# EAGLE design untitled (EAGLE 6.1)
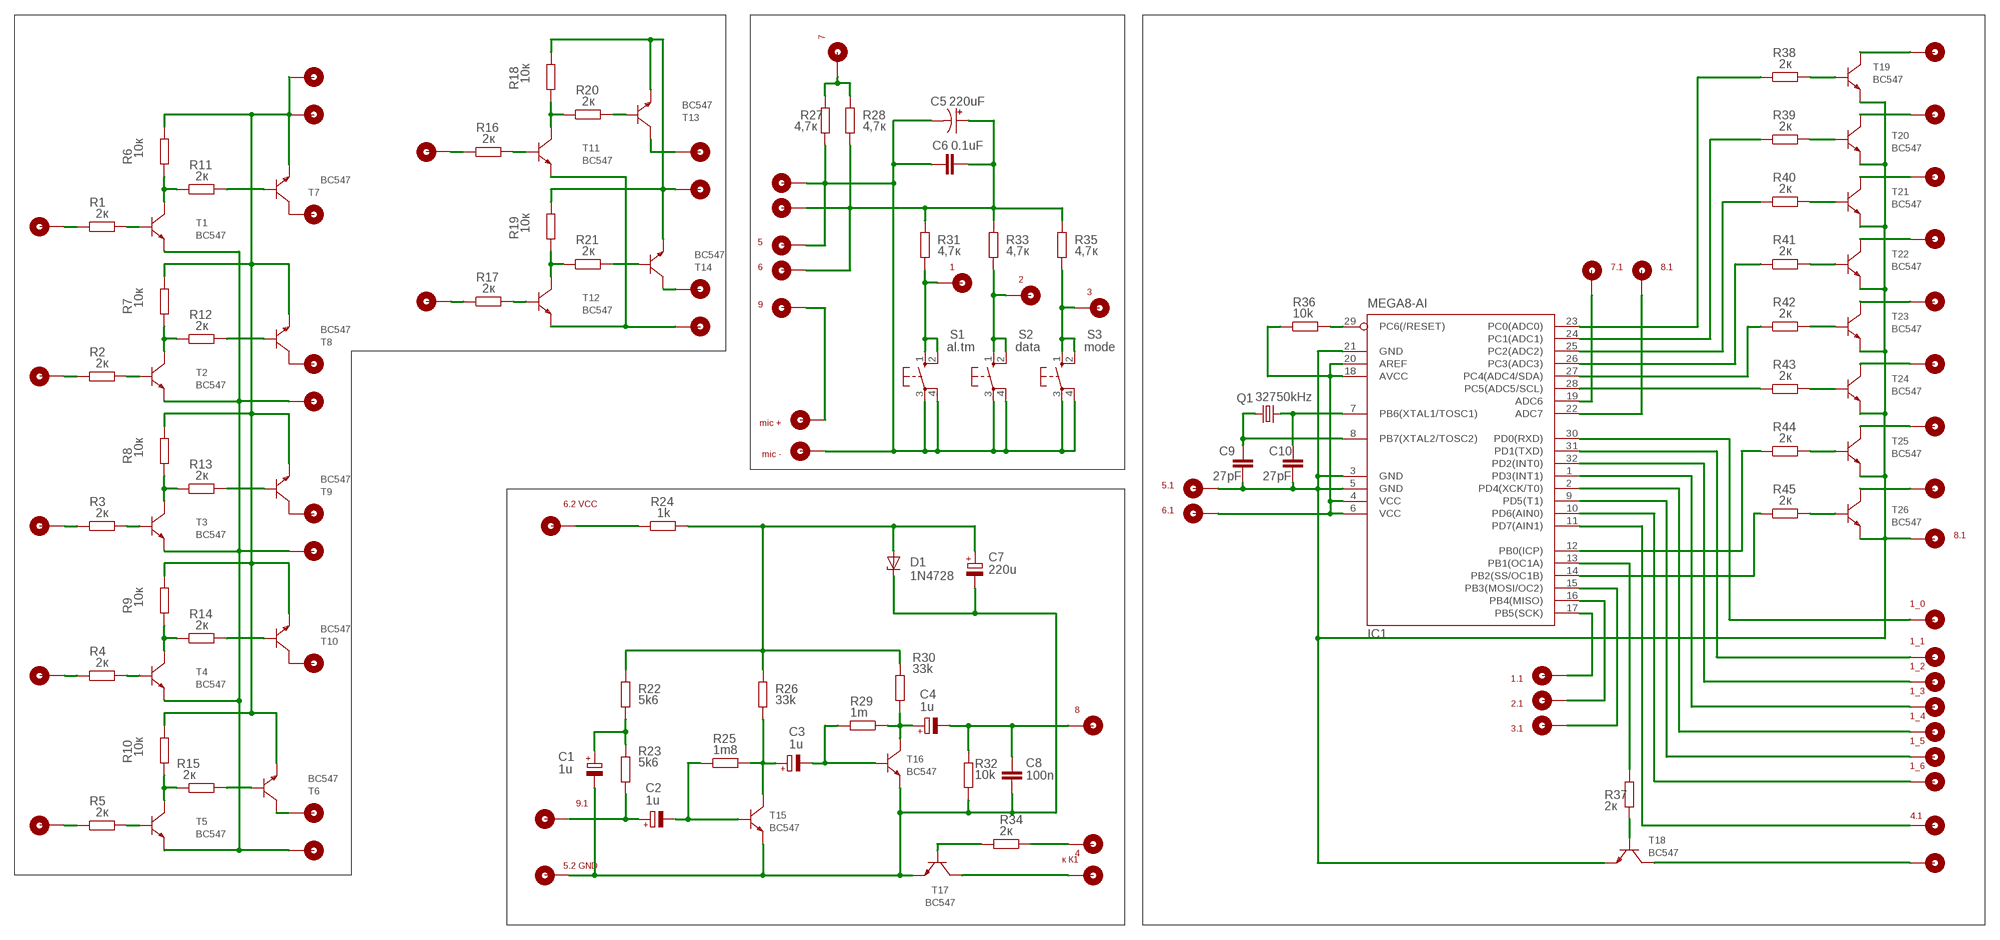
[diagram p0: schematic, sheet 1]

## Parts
1  1_0  PIN_1  [PIN_1]
2  1_1  PIN_1  [PIN_1]
3  1_2  PIN_1  [PIN_1]
C1  1u  CPOL-EUE2.5-6  [E2,5-6]
C2  1u  CPOL-EUE2.5-6  [E2,5-6]
C3  1u  CPOL-EUE2.5-6  [E2,5-6]
C4  1u  CPOL-EUE2.5-6  [E2,5-6]
C5  220uF  CPOL-US153CLV-0810  [153CLV-0810]
C6  0.1uF  C-EU050-024X044  [C050-024X044]
C7  220u  CPOL-EUE3.5-8  [E3,5-8]
C8  100n  C-EU050-024X044  [C050-024X044]
C9  27pF  C-EU050-024X044  [C050-024X044]
C10  27pF  C-EU050-024X044  [C050-024X044]
D1  1N4728  [DO41Z10]
IC1  MEGA8-AI  [TQFP32-08]
Q1  32750kHz  CRYSTALTC38H  [TC38H]
R1  2к  R-EU_0207/10  [0207/10]
R2  2к  R-EU_0207/10  [0207/10]
R3  2к  R-EU_0207/10  [0207/10]
R4  2к  R-EU_0207/10  [0207/10]
R5  2к  R-EU_0207/10  [0207/10]
R6  10к  R-EU_0207/10  [0207/10]
R7  10к  R-EU_0207/10  [0207/10]
R8  10к  R-EU_0207/10  [0207/10]
R9  10к  R-EU_0207/10  [0207/10]
R10  10к  R-EU_0207/10  [0207/10]
R11  2к  R-EU_0207/10  [0207/10]
R12  2к  R-EU_0207/10  [0207/10]
R13  2к  R-EU_0207/10  [0207/10]
R14  2к  R-EU_0207/10  [0207/10]
R15  2к  R-EU_0207/10  [0207/10]
R16  2к  R-EU_0207/10  [0207/10]
R17  2к  R-EU_0207/10  [0207/10]
R18  10к  R-EU_0207/10  [0207/10]
R19  10к  R-EU_0207/10  [0207/10]
R20  2к  R-EU_0207/10  [0207/10]
R21  2к  R-EU_0207/10  [0207/10]
R22  5k6  R-EU_0207/10  [0207/10]
R23  5k6  R-EU_0207/10  [0207/10]
R24  1k  R-EU_0207/10  [0207/10]
R25  1m8  R-EU_0207/10  [0207/10]
R26  33k  R-EU_0207/10  [0207/10]
R27  4,7к  R-EU_0207/10  [0207/10]
R28  4,7к  R-EU_0207/10  [0207/10]
R29  1m  R-EU_0207/10  [0207/10]
R30  33k  R-EU_0207/10  [0207/10]
R31  4,7к  R-EU_0207/10  [0207/10]
R32  10k  R-EU_0207/10  [0207/10]
R33  4,7к  R-EU_0207/10  [0207/10]
R34  2к  R-EU_0207/10  [0207/10]
R35  4,7к  R-EU_0207/10  [0207/10]
R36  10k  R-EU_0207/12  [0207/12]
R37  2к  R-EU_0207/10  [0207/10]
R38  2к  R-EU_0207/10  [0207/10]
R39  2к  R-EU_0207/10  [0207/10]
R40  2к  R-EU_0207/10  [0207/10]
R41  2к  R-EU_0207/10  [0207/10]
R42  2к  R-EU_0207/10  [0207/10]
R43  2к  R-EU_0207/10  [0207/10]
R44  2к  R-EU_0207/10  [0207/10]
R45  2к  R-EU_0207/10  [0207/10]
S1  al.tm  10-XX  [B3F-10XX]
S2  data  10-XX  [B3F-10XX]
S3  mode  10-XX  [B3F-10XX]
T1  BC547  [BC547]
T2  BC547  [BC547]
T3  BC547  [BC547]
T4  BC547  [BC547]
T5  BC547  [BC547]
T6  BC547  [BC547]
T7  BC547  [BC547]
T8  BC547  [BC547]
T9  BC547  [BC547]
T10  BC547  [BC547]
T11  BC547  [BC547]
T12  BC547  [BC547]
T13  BC547  [BC547]
T14  BC547  [BC547]
T15  BC547  [BC547]
T16  BC547  [BC547]
T17  BC547  [BC547]
T18  BC547  [BC547]
T19  BC547  [BC547]
T20  BC547  [BC547]
T21  BC547  [BC547]
T22  BC547  [BC547]
T23  BC547  [BC547]
T24  BC547  [BC547]
T25  BC547  [BC547]
T26  BC547  [BC547]
U$1  PIN_1  [PIN_1]
U$2  PIN_1  [PIN_1]
U$3  PIN_1  [PIN_1]
U$4  PIN_1  [PIN_1]
U$5  PIN_1  [PIN_1]
U$6  PIN_1  [PIN_1]
U$7  PIN_1  [PIN_1]
U$8  PIN_1  [PIN_1]
U$9  PIN_1  [PIN_1]
U$10  PIN_1  [PIN_1]
U$11  PIN_1  [PIN_1]
U$12  PIN_1  [PIN_1]
U$13  PIN_1  [PIN_1]
U$14  PIN_1  [PIN_1]
U$15  PIN_1  [PIN_1]
U$16  PIN_1  [PIN_1]
U$17  PIN_1  [PIN_1]
U$18  9.1  PIN_1  [PIN_1]
U$19  5.2 GND  PIN_1  [PIN_1]
U$20  6.2 VCC  PIN_1  [PIN_1]
U$21  PIN_1  [PIN_1]
U$22  PIN_1  [PIN_1]
U$23  PIN_1  [PIN_1]
U$24  PIN_1  [PIN_1]
U$25  PIN_1  [PIN_1]
U$26  PIN_1  [PIN_1]
U$27  5  PIN_1  [PIN_1]
U$28  6  PIN_1  [PIN_1]
U$29  9  PIN_1  [PIN_1]
U$30  mic +  PIN_1  [PIN_1]
U$31  mic -  PIN_1  [PIN_1]
U$32  7  PIN_1  [PIN_1]
U$33  1  PIN_1  [PIN_1]
U$34  2  PIN_1  [PIN_1]
U$35  8  PIN_1  [PIN_1]
U$36  4  PIN_1  [PIN_1]
U$37  к К1  PIN_1  [PIN_1]
U$38  3  PIN_1  [PIN_1]
U$39  5.1  PIN_1  [PIN_1]
U$40  6.1  PIN_1  [PIN_1]
U$41  1.1  PIN_1  [PIN_1]
U$42  2.1  PIN_1  [PIN_1]
U$43  3.1  PIN_1  [PIN_1]
U$44  7.1  PIN_1  [PIN_1]
U$45  8.1  PIN_1  [PIN_1]
U$46  PIN_1  [PIN_1]
U$47  PIN_1  [PIN_1]
U$48  PIN_1  [PIN_1]
U$49  PIN_1  [PIN_1]
U$50  PIN_1  [PIN_1]
U$51  PIN_1  [PIN_1]
U$52  PIN_1  [PIN_1]
U$53  PIN_1  [PIN_1]
U$54  8.1  PIN_1  [PIN_1]
U$55  1_3  PIN_1  [PIN_1]
U$56  1_4  PIN_1  [PIN_1]
U$57  1_5  PIN_1  [PIN_1]
U$58  1_6  PIN_1  [PIN_1]
U$59  4.1  PIN_1  [PIN_1]
U$60  PIN_1  [PIN_1]

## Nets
GND: C5.- C6.2 R27.1 S1.3(P) S1.4(P1) S2.3(P) S2.4(P1) S3.3(P) S3.4(P1) U$25.P$1 U$27.P$1 U$31.P$1
N$1: R42.2 T23.B
N$2: 2.P$1 IC1.31(PD1(TXD))
N$7: R31.1 S1.1(S) S1.2(S1) U$33.P$1
N$8: R27.2 R28.2 U$32.P$1
N$9: IC1.28(PC5(ADC5/SCL)) R43.1
N$10: IC1.27(PC4(ADC4/SDA)) R42.1
N$11: IC1.26(PC3(ADC3)) R41.1
N$12: IC1.25(PC2(ADC2)) R40.1
N$13: IC1.24(PC1(ADC1)) R39.1
N$14: IC1.23(PC0(ADC0)) R38.1
N$15: C9.2 C10.2 IC1.3(GND) IC1.5(GND) IC1.21(GND) T18.E T19.E T20.E T21.E T22.E T23.E T24.E T25.E T26.E U$39.P$1 U$54.P$1
N$16: IC1.14(PB2(SS/OC1B)) R45.1
N$17: R43.2 T24.B
N$18: R33.1 S2.1(S) S2.2(S1) U$34.P$1
N$19: IC1.12(PB0(ICP)) R44.1
N$20: R41.2 T22.B
N$21: R40.2 T21.B
N$22: R39.2 T20.B
N$23: R38.2 T19.B
N$24: R45.2 T26.B
N$25: R44.2 T25.B
N$26: T25.K U$52.P$1
N$27: T26.K U$53.P$1
N$28: T19.K U$46.P$1
N$29: T20.K U$47.P$1
N$30: T21.K U$48.P$1
N$31: T22.K U$49.P$1
N$32: T23.K U$50.P$1
N$33: T24.K U$51.P$1
N$34: 1.P$1 IC1.30(PD0(RXD))
N$35: R35.1 S3.1(S) S3.2(S1) U$38.P$1
N$36: 3.P$1 IC1.32(PD2(INT0))
N$37: IC1.1(PD3(INT1)) U$55.P$1
N$38: IC1.2(PD4(XCK/T0)) U$56.P$1
N$39: IC1.9(PD5(T1)) U$57.P$1
N$40: IC1.10(PD6(AIN0)) U$58.P$1
N$41: C9.1 IC1.8(PB7(XTAL2/TOSC2)) Q1.1
N$42: IC1.17(PB5(SCK)) U$41.P$1
N$43: IC1.16(PB4(MISO)) U$42.P$1
N$44: IC1.15(PB3(MOSI/OC2)) U$43.P$1
N$45: IC1.13(PB1(OC1A)) R37.1
N$46: IC1.4(VCC) IC1.6(VCC) IC1.18(AVCC) IC1.20(AREF) R36.1 U$40.P$1
N$47: C10.1 IC1.7(PB6(XTAL1/TOSC1)) Q1.2
N$48: IC1.29(PC6(/RESET)) R36.2
N$49: T18.K U$60.P$1
N$50: IC1.19(ADC6) U$44.P$1
N$51: IC1.11(PD7(AIN1)) U$59.P$1
N$52: IC1.22(ADC7) U$45.P$1
N$53: R37.2 T18.B
N$56: C5.+ C6.1 R28.1 R31.2 R33.2 R35.2 U$26.P$1 U$28.P$1
N$57: R34.1 U$36.P$1
N$63: C4.- C8.2 R32.2 U$35.P$1
N$75: C4.+ R29.1 R30.1 T16.K
N$77: R1.1 U$1.P$1
N$78: R1.2 T1.B
N$79: T11.E T12.E U$24.P$1
N$80: R6.1 R11.1 T1.K
N$81: T7.K U$8.P$1
N$82: R2.1 U$2.P$1
N$83: R2.2 T2.B
N$85: R7.1 R12.1 T2.K
N$86: T8.K U$9.P$1
N$87: R3.1 U$3.P$1
N$88: R3.2 T3.B
N$90: R8.1 R13.1 T3.K
N$91: T9.K U$11.P$1
N$92: R4.1 U$4.P$1
N$93: R4.2 T4.B
N$95: R9.1 R14.1 T4.K
N$96: T10.K U$13.P$1
N$97: R5.1 U$5.P$1
N$98: R5.2 T5.B
N$99: R6.2 R7.2 R8.2 R9.2 R10.2 T6.E T7.E T8.E T9.E T10.E U$6.P$1 U$7.P$1
N$128: R34.2 T17.B
N$129: C3.- R29.2 T16.B
N$130: C3.+ R25.2 R26.2 T15.K
N$131: C2.- R25.1 T15.B
N$132: C2.+ R23.2 U$18.P$1
N$136: U$29.P$1 U$30.P$1
N$139: C1.+ R22.2 R23.1
N$141: C7.+ D1.A R22.1 R24.2 R26.1 R30.2
N$143: C1.- C7.- C8.1 D1.C R32.1 T15.E T16.E T17.E U$19.P$1
N$146: R24.1 U$20.P$1
N$149: T17.K U$37.P$1
N$184: R10.1 R15.1 T5.K
N$185: T6.K U$14.P$1
N$186: R16.1 U$16.P$1
N$187: R16.2 T11.B
N$189: R18.1 R20.1 T11.K
N$190: T13.K U$21.P$1
N$191: R17.1 U$17.P$1
N$192: R17.2 T12.B
N$193: R18.2 R19.2 T13.E T14.E U$22.P$1
N$194: R19.1 R21.1 T12.K
N$195: T14.K U$23.P$1
N$196: T1.E T2.E T3.E T4.E T5.E U$10.P$1 U$12.P$1 U$15.P$1
N$340: R15.2 T6.B
N$341: R14.2 T10.B
N$342: R13.2 T9.B
N$343: R11.2 T7.B
N$344: R12.2 T8.B
N$345: R21.2 T14.B
N$346: R20.2 T13.B

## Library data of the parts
1-3 U$1-U$60 = untitled:PIN_1
C1-C4 C7 = rcl:CPOL-EU: POLARIZED CAPACITOR, European symbol
C5 = rcl:CPOL-US: POLARIZED CAPACITOR, American symbol
C6 C8-C10 = rcl:C-EU: CAPACITOR, European symbol
D1 = diode:1N4728: Z DIODE
IC1 = atmel:MEGA8: MICROCONTROLLER 8 Kbytes FLASH, 1 kbytes SRAM, 512 bytes EEPROM, USART, 6-channel 10 bit ADC, 2-channel 8 bit ADC Pin compatible with Atmega48, ATMega88, ATMega168 Source: avr.lbr; MPN: ATMEGA8-16AU; OC_FARNELL: 9171371; OC_NEWARK: 73M8863
Q1 = crystal:CRYSTAL: CRYSTAL; OC_FARNELL: unknown; OC_NEWARK: unknown
R1-R45 = rcl:R-EU_: RESISTOR, European symbol
S1-S3 = switch-omron:10-XX: OMRON SWITCH; MPN: B3F-1000; OC_FARNELL: 176432; OC_NEWARK: 36M3542
T1-T26 = untitled:BC547

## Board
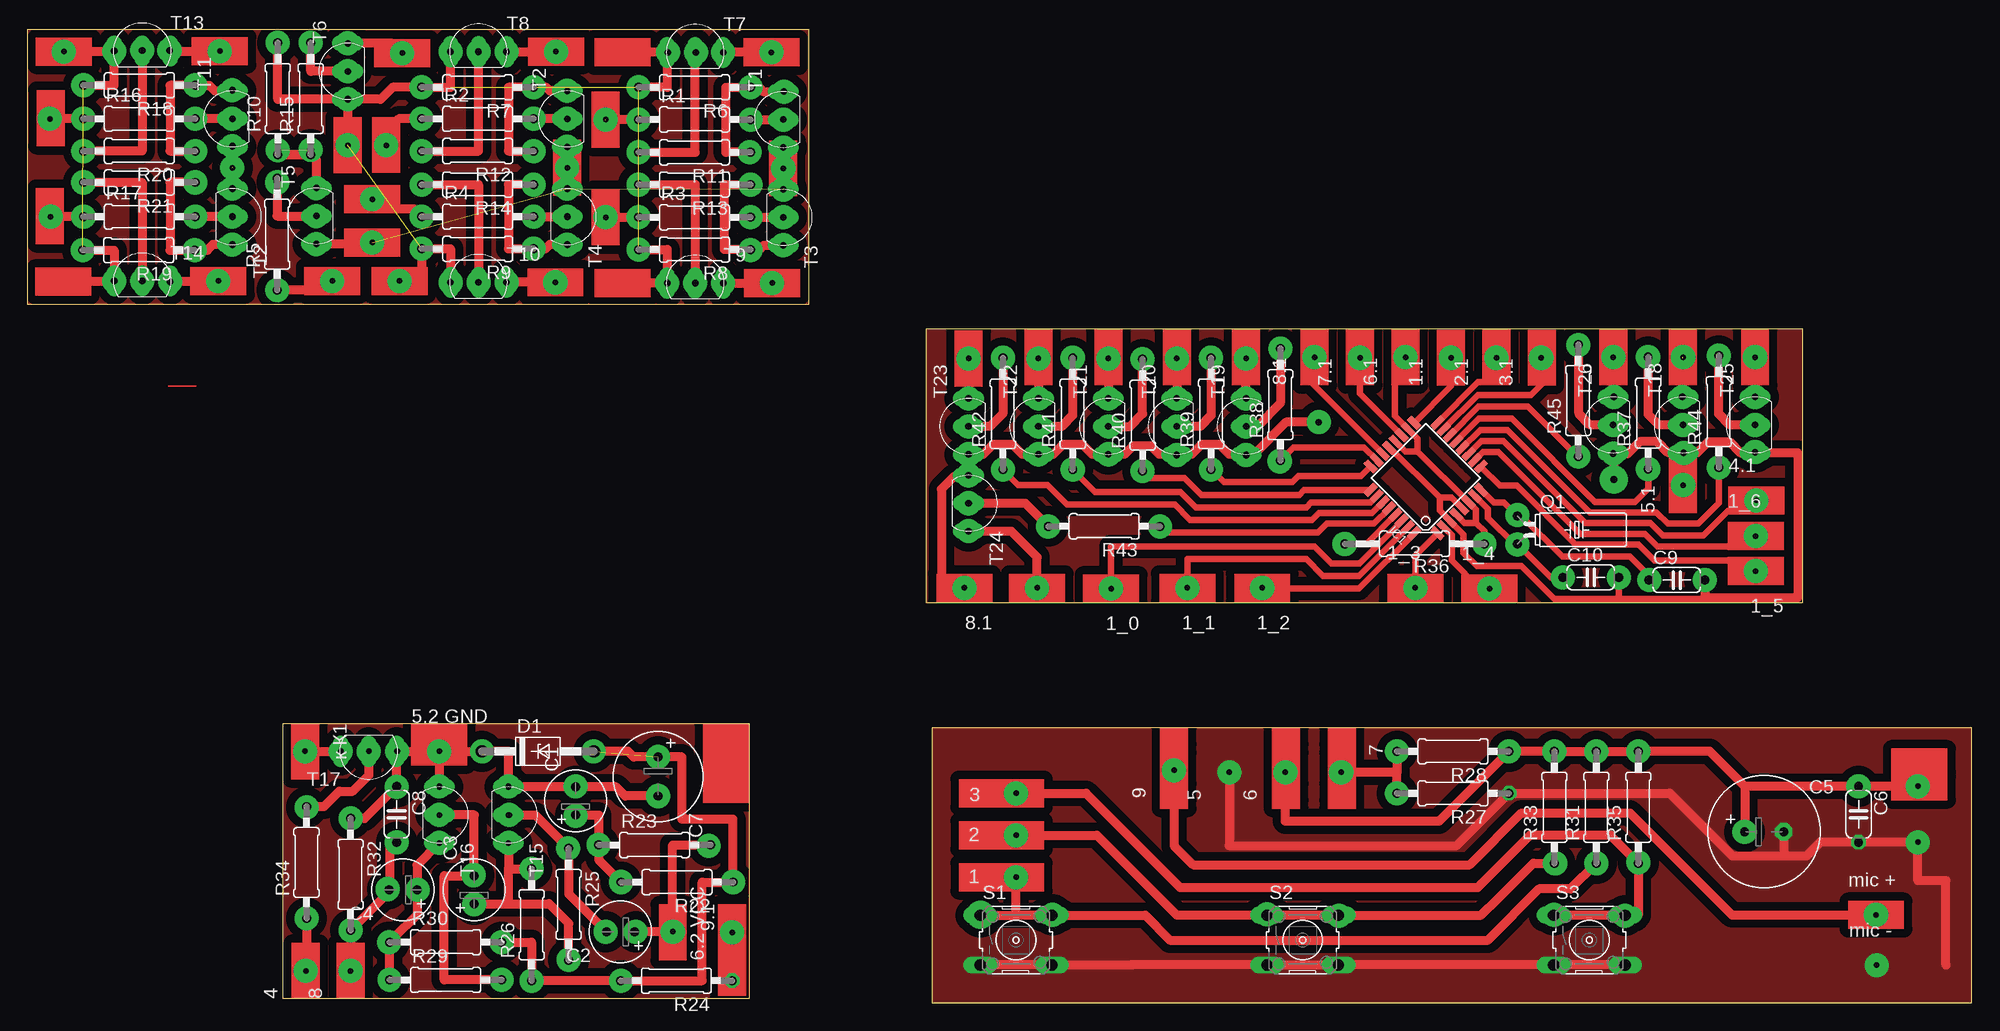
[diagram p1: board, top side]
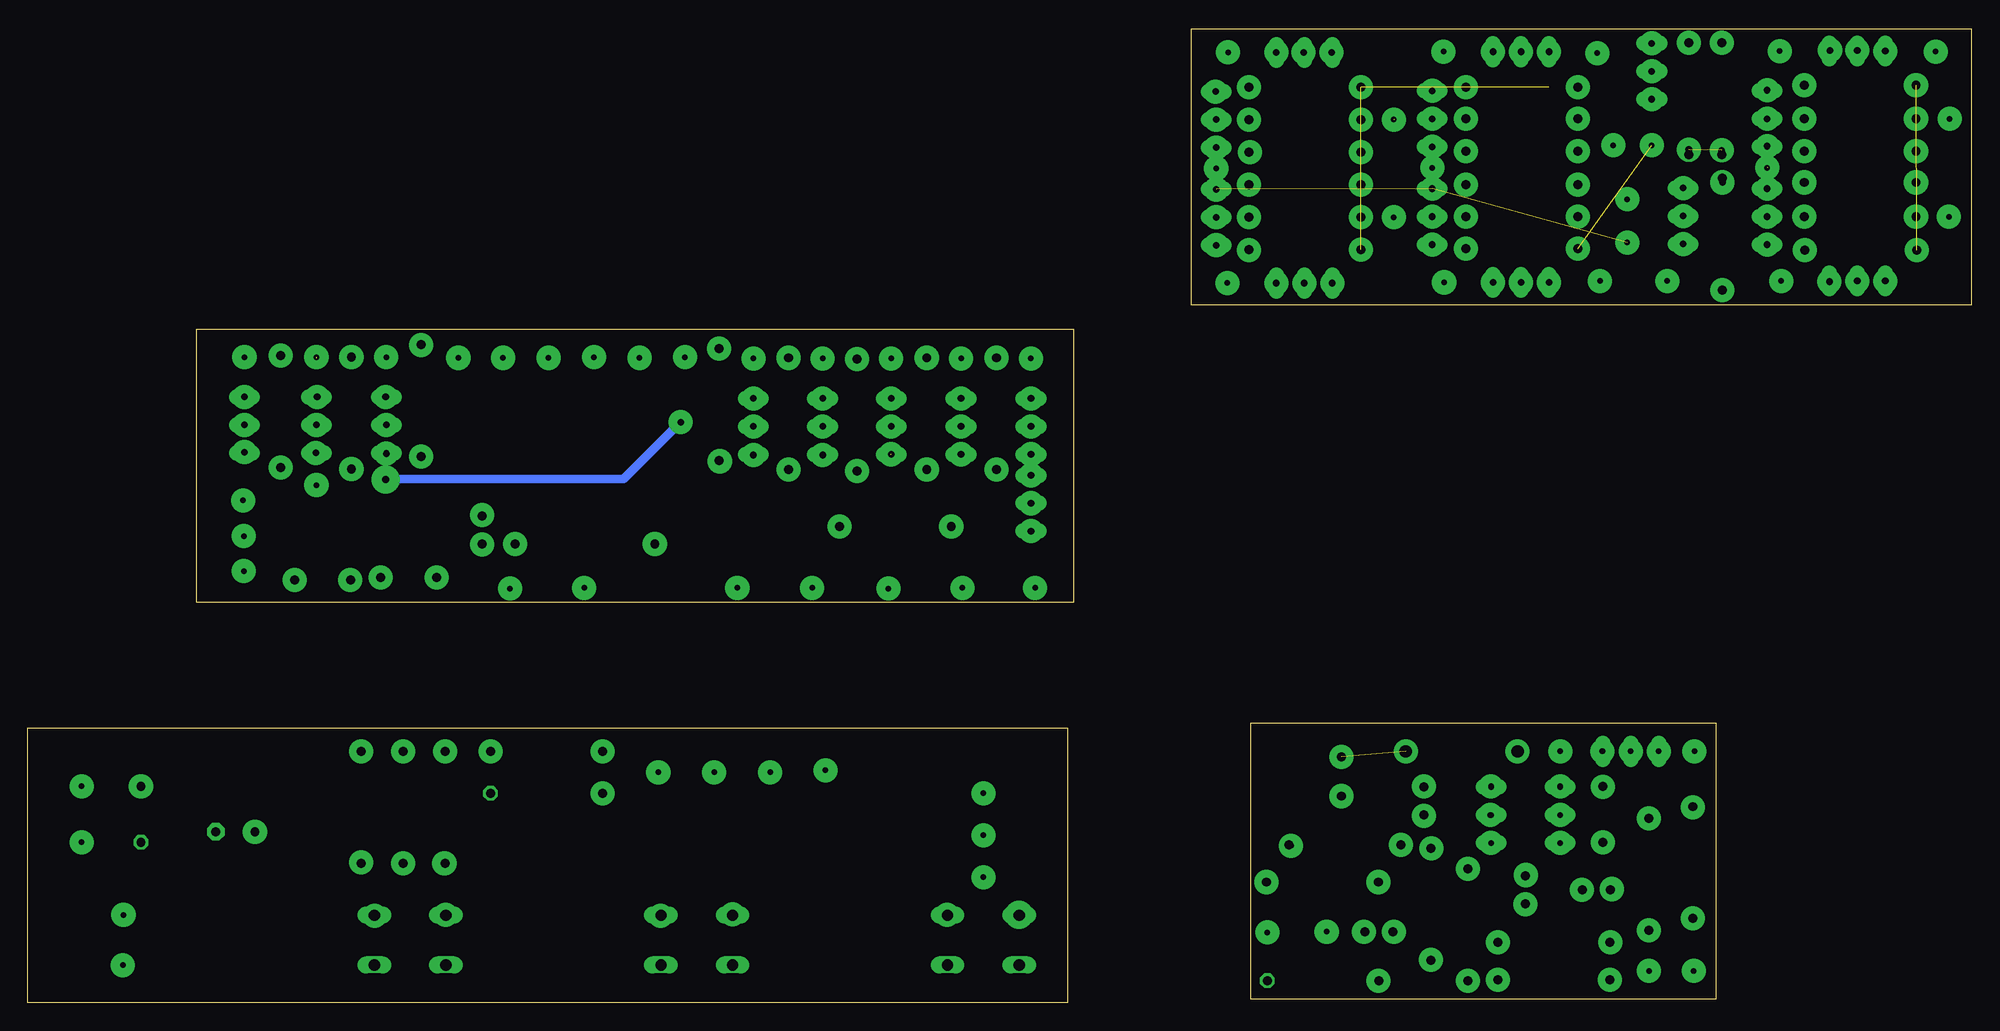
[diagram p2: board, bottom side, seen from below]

Size 176.61 x 88.46 mm. Coordinates in mm from the lower left corner, seen from the top.
Outline: 82.17,0 176.61,0 176.61,25 82.17,25 82.17,0
Outline: 81.6,36.39 161.23,36.39 161.23,61.21 81.6,61.21 81.6,36.39
Outline: 65.53,25.4 65.53,0.38 23.24,0.38 23.24,25.4 65.53,25.4
Outline: 70.93,88.46 70.93,63.44 0,63.44 0,88.46 70.93,88.46
Copper layers (1*16): Top 0.035mm / dielectric 1.5mm / Bottom 0.035mm
Design rules: minimum track width 10mil, minimum drill 24mil, track to track 30mil, track to pad 25mil, pad to pad 8mil, via to via 8mil, smd to smd 8mil, copper to edge 0mil, drill to drill 8mil, minimum pad ring 10mil, minimum via ring 8mil, stop-mask expansion 4mil, vias tented up to drill 0mil, thermal gap 0mil

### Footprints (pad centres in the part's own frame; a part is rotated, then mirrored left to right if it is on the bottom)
PIN_1 = drill 0.5 pad 2.184: P$1 0,0
E2,5-6 = drill 0.813 pad 1.6: + -1.27,0 | drill 0.813 pad 1.6 octagon: - 1.27,0
E3,5-10 = drill 0.813 pad 1.6: + -1.778,0 | drill 0.813 pad 1.6 octagon: - 1.778,0
C050-024X044 = drill 0.813 octagon: 1 -2.54,0; 2 2.54,0
E3,5-8 = drill 0.813 pad 1.6: + -1.778,0 | drill 0.813 pad 1.6 octagon: - 1.778,0
DO41Z10 = drill 1.118: A 5.08,0; C -5.08,0
TQFP32-08 = smd 1.27 x 0.559: 1 -4.293,2.8; 2 -4.293,2; 3 -4.293,1.2; 4 -4.293,0.4; 5 -4.293,-0.4; 6 -4.293,-1.2; 7 -4.293,-2; 8 -4.293,-2.8; 17 4.293,-2.8; 18 4.293,-2; 19 4.293,-1.2; 20 4.293,-0.4; 21 4.293,0.4; 22 4.293,1.2; 23 4.293,2; 24 4.293,2.8 | smd 0.559 x 1.27: 9 -2.8,-4.293; 10 -2,-4.293; 11 -1.2,-4.293; 12 -0.4,-4.293; 13 0.4,-4.293; 14 1.2,-4.293; 15 2,-4.293; 16 2.8,-4.293; 25 2.8,4.293; 26 2,4.293; 27 1.2,4.293; 28 0.4,4.293; 29 -0.4,4.293; 30 -1.2,4.293; 31 -2,4.293; 32 -2.8,4.293
TC38H = drill 0.813: 1 -1.27,0; 2 1.27,0
0207/10 = drill 0.813 octagon: 1 -5.08,0; 2 5.08,0
0207/12 = drill 0.813 octagon: 1 -6.35,0; 2 6.35,0
B3F-10XX = drill 1.016 long: 1 -3.251,2.261; 2 3.251,2.261; 3 -3.251,-2.261; 4 3.251,-2.261
BC547 = drill 0.5 pad 1.422 long: B 0,0; E -2.54,0; K 2.54,0

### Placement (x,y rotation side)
1  98.42,37.66 180 top
2  105.35,37.72 180 top
3  112.14,37.72 180 top
C1  49.78,18.35 90 top
C2  53.85,6.48 180 top
C3  40.58,10.29 90 top
C4  34.1,10.29 180 top
C5  220uF  [E3,5-10]  157.73,15.56 0 top
C6  166.31,17.14 270 top
C7  57.28,20.57 270 top
C8  33.53,17.14 270 top
C9  149.8,38.42 0 top
C10  141.99,38.67 0 top
D1  46.36,22.86 0 top
IC1  127,47.69 135 top
Q1  135.32,42.99 270 top
R1  60.58,80.26 0 top
R2  40.89,80.33 0 top
R3  60.58,71.37 0 top
R4  40.89,71.44 0 top
R5  22.67,69.85 90 top
R6  60.58,83.19 180 top
R7  40.89,83.19 180 top
R8  60.58,68.45 180 top
R9  40.89,68.52 180 top
R10  22.73,82.17 90 top
R11  60.58,77.28 180 top
R12  40.89,77.41 180 top
R13  60.58,74.36 180 top
R14  40.89,74.36 180 top
R15  25.72,82.17 90 top
R16  10.16,80.33 0 top
R17  10.16,71.44 0 top
R18  10.16,83.38 180 top
R19  10.1,68.39 180 top
R20  10.16,77.41 180 top
R21  10.16,74.55 180 top
R22  58.99,10.99 180 top
R23  56.96,14.35 0 top
R24  58.93,2.03 180 top
R25  49.15,8.95 270 top
R26  45.78,7.11 90 top
R27  129.48,19.05 180 top
R28  129.48,22.86 180 top
R29  37.97,2.1 0 top
R30  37.97,5.52 0 top
R31  142.49,17.78 90 top
R32  29.34,11.68 270 top
R33  138.68,17.78 90 top
R34  25.34,12.76 90 top
R35  146.3,17.78 90 top
R36  125.98,41.72 180 top
R37  147.19,53.59 90 top
R38  113.79,54.36 90 top
R39  107.51,53.53 90 top
R40  101.28,53.4 90 top
R41  94.93,53.53 90 top
R42  88.58,53.53 90 top
R43  97.79,43.31 180 top
R44  153.61,53.72 90 top
R45  140.84,54.74 90 top
S1  89.79,5.72 0 top
S2  115.82,5.72 0 top
S3  141.86,5.72 0 top
T1  68.64,80.26 90 top
T2  49.02,80.33 90 top
T3  68.64,71.37 270 top
T4  49.02,71.44 270 top
T5  26.23,71.5 90 top
T6  29.08,84.65 90 top
T7  60.64,86.36 0 top
T8  40.96,86.42 0 top
T9  60.64,65.41 0 top
T10  40.96,65.47 0 top
T11  18.61,80.33 90 top
T12  18.61,71.44 270 top
T13  10.41,86.49 0 top
T14  10.41,65.6 0 top
T15  43.69,17.08 270 top
T16  37.4,17.08 270 top
T17  30.99,22.86 180 top
T18  150.37,52.51 90 top
T19  110.68,52.39 90 top
T20  104.39,52.39 90 top
T21  98.17,52.39 90 top
T22  91.82,52.39 90 top
T23  85.47,52.39 90 top
T24  85.47,45.4 270 top
T25  156.91,52.51 90 top
T26  144.02,52.51 90 top
U$1  52.51,80.26 90 top
U$2  32.58,77.91 270 top
U$3  52.51,71.37 90 top
U$4  31.31,73.03 180 top
U$5  27.69,65.6 180 top
U$6  29.08,77.91 270 top
U$7  33.78,65.6 0 top
U$8  67.56,86.36 180 top
U$9  48.01,86.42 180 top
U$10  49.02,75.88 90 top
U$11  67.63,65.41 0 top
U$12  68.64,75.82 90 top
U$13  47.94,65.47 0 top
U$14  34.04,86.3 180 top
U$15  31.31,69.09 180 top
U$16  2.03,80.33 90 top
U$17  2.1,71.44 90 top
U$18  58.61,6.48 270 top
U$19  37.4,22.86 0 top
U$20  64.01,6.41 90 top
U$21  17.46,86.49 0 top
U$22  3.3,86.42 180 top
U$23  17.34,65.6 0 top
U$24  18.61,75.88 90 top
U$25  171.7,14.6 180 top
U$26  171.7,19.69 180 top
U$27  109.16,20.96 90 top
U$28  114.24,20.96 90 top
U$29  104.14,21.15 90 top
U$30  167.89,8 0 top
U$31  167.96,3.43 0 top
U$32  119.32,20.96 270 top
U$33  89.79,11.43 0 top
U$34  89.79,15.24 0 top
U$35  29.34,2.92 90 top
U$36  25.27,2.92 90 top
U$37  25.21,22.86 270 top
U$38  89.79,19.05 0 top
U$39  150.37,47.05 90 top
U$40  125.16,58.67 90 top
U$41  129.29,58.61 90 top
U$42  133.41,58.61 90 top
U$43  137.48,58.61 90 top
U$44  121.03,58.61 90 top
U$45  116.9,58.67 90 top
U$46  110.68,58.55 90 top
U$47  104.39,58.55 90 top
U$48  98.17,58.55 90 top
U$49  91.82,58.55 90 top
U$50  85.47,58.55 90 top
U$51  91.69,37.72 0 top
U$52  156.91,58.67 90 top
U$53  144.02,58.67 90 top
U$54  85.09,37.72 180 top
U$55  126.05,37.72 0 top
U$56  132.78,37.66 0 top
U$57  156.97,39.24 180 top
U$58  156.97,42.42 0 top
U$59  157.04,45.66 0 top
U$60  150.37,58.67 90 top

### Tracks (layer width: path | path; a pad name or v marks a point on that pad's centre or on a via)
GND
  Top 0.813: 174.24,3.45 174.24,11.11 171.7,11.11 U$25.P$1 C6.2 162.81,14.6 161.54,13.33 159.32,13.33 | S3.4 S3.3 S2.4 S2.3 100.31,3.45 arc-90 100.27,3.49 arc-90 100.23,3.45 S1.4 S1.3 | U$27.P$1 109.16,14.29 129.79,14.29 R27.1 149.16,19.05 154.88,13.33 159.32,13.33 | C5.- 159.51,13.53 159.32,13.33
  pour Top: 176.47,25.08 176.47,0 82.17,0 82.17,25.02 86.23,25.02
GND1
  pour Top: 81.6,61.21 81.6,36.45 161.23,36.45 161.23,61.21
N$1
  Top 0.813: R42.2 88.58,53.53 87.44,52.39 T23.B
N$2
  Top 0.61: IC1.31 120.94,38.8 117.67,38.8 116.14,40.32 105.35,40.32 2.P$1
N$3  (via drill 0.6 pad 2.18)
  other vias: 22.67,64.77
N$4  (via drill 0.6 pad 2.18)
  other vias: 18.61,73.98
N$5  (via drill 0.6 pad 2.18)
  other vias: 26.23,68.96
N$6  (via drill 0.6 pad 2.18)
  other vias: 26.23,71.5
N$7
  Top 0.813: R31.1 140.14,10.35 137.29,10.35 132.65,5.72 103.76,5.72 101.54,7.98 S1.2 89.79,7.98 | 89.79,7.98 U$33.P$1 | S1.1 89.79,7.98
N$8
  Top 0.813: R27.2 124.4,20.96 | 124.4,20.96 U$32.P$1 | R28.2 124.4,20.96
N$9
  Top 0.61: IC1.28 122.3,43.56 118.04,43.56 117.22,42.74 103.5,42.74 R43.1
N$10
  Top 0.61: IC1.27 122.13,44.51 117.28,44.51 116.65,43.88 105.6,43.88 104.2,45.28 94.42,45.28 92.65,47.05 89.98,47.05 R42.1
N$11
  Top 0.61: IC1.26 121.95,45.47 116.59,45.47 116.14,45.02 106.11,45.02 104.71,46.42 96.96,46.42 R41.1
N$12
  Top 0.61: IC1.25 121.95,46.61 115.95,46.61 115.51,46.16 106.62,46.16 105.09,47.69 101.92,47.69 R40.1
N$13
  Top 0.61: IC1.24 121.12,47.88 115.44,47.88 114.87,47.31 108.65,47.31 R39.1
N$14
  Top 0.61: IC1.23 121.38,50.48 115,50.48 R38.1
N$15  (via drill 0.6, 0.6 pad 2.18, 0.6 pad 2.54)  (1 unrouted)
  Top 0.61: IC1.5 129.34,45.91 128.27,45.91 | 128.27,45.91 128.27,44.72 IC1.3 130.43,42.56 130.43,40.89 131.64,39.69 135.7,39.69 138.68,36.7 144.53,36.7 | 128.27,45.91 IC1.21 | C9.2 152.34,36.7 144.53,36.7 | 144.53,36.7 C10.2 | U$39.P$1 T18.E
  Top 0.813: 98.23,49.85 99.63,49.85 100.39,50.61 102.04,50.61 102.81,49.85 T20.E 105.73,49.85 106.62,50.74 108.27,50.74 109.16,49.85 T19.E 111.38,49.85 114.3,52.77 v117.28,52.77 | T21.E 96.71,49.85 95.82,50.74 94.04,50.74 93.15,49.85 T22.E | T22.E 91.76,49.85 | T22.E 90.36,49.85 89.47,50.74 87.69,50.74 86.81,49.85 T23.E T24.E 84.14,47.82 83,46.67 83,37.72 U$54.P$1 | T26.E 144.08,49.91 | 144.08,49.91 v144.08,47.56 | C9.2 152.34,36.83 160.78,36.83 160.78,49.97 T25.E 155.57,49.97 154.56,50.99 152.65,50.99 151.64,49.97 T18.E 149.03,49.97 148.02,50.99 146.43,50.99 145.35,49.91 144.08,49.91
  Bottom 0.813: v144.08,47.56 122.49,47.63 v117.28,52.77
  other vias: 152.34,38.42
N$16
  Top 0.61: IC1.14 131.78,54.17 136.27,54.17 140.78,49.66 R45.1
N$17
  Top 0.813: T24.B 90.61,45.4 R43.2
N$18
  Top 0.813: R33.1 136.78,12.7 133.6,9.52 132.02,7.98 S2.2 S2.1 104.39,7.98 97.13,15.24 U$34.P$1
N$19
  Top 0.61: R44.1 153.61,45.4 151.76,43.56 148.97,43.56 147.95,44.58 141.92,44.58 134.43,52.07 131.95,52.07 IC1.12
N$20
  Top 0.813: R41.2 94.93,53.4 93.92,52.39 T22.B
N$21
  Top 0.813: T21.B 100.14,52.39 101.28,53.53 R40.2
N$22
  Top 0.813: R39.2 107.5,53.4 106.49,52.39 T20.B
N$23
  Top 0.813: T19.B 111.7,52.39 113.79,54.48 R38.2
N$24
  Top 0.813: T26.B 141.92,52.51 140.91,53.53 140.91,59.75 R45.2
N$25
  Top 0.813: T25.B 154.62,52.51 153.61,53.53 R44.2
N$26
  Top 0.813: U$52.P$1 T25.K
N$27
  Top 0.813: T26.K U$53.P$1
N$28
  Top 0.813: T19.K U$46.P$1
N$29
  Top 0.813: U$47.P$1 T20.K
N$30
  Top 0.813: U$48.P$1 T21.K
N$31
  Top 0.813: U$49.P$1 T22.K
N$32
  Top 0.813: U$50.P$1 T23.K
N$33
  Top 0.813: T24.K 89.34,42.86 91.69,40.51 U$51.P$1
N$34
  Top 0.61: IC1.30 120.95,39.94 118.43,39.94 116.9,41.47 98.42,41.47 1.P$1
N$35
  Top 0.813: S3.1 S3.2 146.3,7.98 R35.1 143.76,15.24 136.46,15.24 131.7,10.48 104.71,10.48 96.14,19.05 U$38.P$1
N$36
  Top 0.61: IC1.32 120.93,37.66 112.2,37.66 3.P$1
N$37
  Top 0.61: IC1.1 126.05,40.67 U$55.P$1
N$38
  Top 0.61: IC1.2 129.35,42.51 129.35,40.2 131.89,37.66 U$56.P$1
N$39
  Top 0.61: IC1.9 132.02,48.68 133.73,46.99 135.25,46.99 140.59,41.66 146.3,41.66 147.76,40.2 156.65,40.2 U$57.P$1
N$40
  Top 0.61: IC1.10 132.18,50.04 133.6,50.04 141.03,42.61 146.88,42.61 148.02,41.47 155.76,41.47 U$58.P$1
N$41
  Top 0.61: IC1.8 133.18,45.47 134.11,45.47 Q1.1 135.7,44.26 139.38,40.58 145.54,40.58 147.26,38.86 C9.1
N$42
  Top 0.61: IC1.17 129.29,56.05 U$41.P$1
N$43
  Top 0.61: IC1.16 131.74,56.39 133.41,56.39 U$42.P$1
N$44
  Top 0.61: U$43.P$1 137.48,56.2 136.53,55.24 131.73,55.24 IC1.15
N$45
  Top 0.61: IC1.13 131.83,53.09 134.81,53.09 142.37,45.53 145.99,45.53 147.19,46.74 R37.1
N$46
  Top 0.61: 126.24,50.1 126.24,51.28 IC1.18 124.21,53.31 124.21,57.02 125.16,57.15 U$40.P$1 | IC1.20 125.15,50.1 126.24,50.1 | 126.24,50.1 IC1.6 131.57,44.81 131.57,43.62 | IC1.4 130.5,43.62 131.57,43.62 | R36.1 132.33,42.86 131.57,43.62
N$47
  Top 0.61: IC1.7 132.65,44.87 132.65,44.07 135.13,41.59 Q1.2 138.37,38.67 C10.1
N$48
  Top 0.61: R36.2 121.6,41.72 IC1.29
N$49  (1 unrouted)
  Top 0.813: T18.K 150.37,58.61
N$50
  Top 0.61: U$44.P$1 121.03,55.35 IC1.19
N$51
  Top 0.61: IC1.11 132.06,51.05 134.05,51.05 141.48,43.62 147.38,43.62 148.53,42.48 152.21,42.48 154.43,44.7 156.65,44.7 U$59.P$1
N$52
  Top 0.61: IC1.22 116.84,56.15 U$45.P$1
N$53
  Top 0.813: T18.B 148.15,52.51 147.19,53.47 R37.2
N$54
  pour Top: 82.17,25.02 82.17,0 176.53,0 176.53,25.02
N$55  (via drill 0.6 pad 2.18)
  other vias: 26.23,74.04
N$56
  Top 0.813: U$26.P$1 C6.1 155.96,19.69 | 155.96,19.69 152.78,22.86 R35.2 R31.2 R33.2 R28.1 128.21,16.51 114.24,16.51 U$28.P$1 | 155.96,19.69 C5.+
N$57
  Top 0.813: R34.1 25.34,2.98 U$36.P$1
N$58  (via drill 0.6 pad 2.18)
  other vias: 22.67,74.55
N$59  (via drill 0.6 pad 2.18)  (1 unrouted)
  other vias: 25.72,77.53 22.73,77.47
N$60  (via drill 0.6 pad 2.18)
  other vias: 29.08,84.65
N$61  (via drill 0.6 pad 2.18)
  other vias: 29.08,82.11
N$62  (via drill 0.6 pad 2.18)
  other vias: 29.08,87.19
N$63
  Top 0.813: C8.2 32.89,13.97 32.89,10.35 C4.- 32.83,10.1 R32.2 U$35.P$1
N$64  (via drill 0.6 pad 2.18)
  other vias: 22.73,87.25
N$65  (via drill 0.6 pad 2.18)
  other vias: 15.24,74.55
N$66
  Top 0.813: 7.87,65.53 4.89,65.53
N$67  (via drill 0.6 pad 2.18)
  other vias: 18.61,68.9
N$68  (via drill 0.6 pad 2.18)
  other vias: 18.61,71.44
N$69  (via drill 0.6 pad 2.18)
  other vias: 5.08,71.44
N$75
  Top 0.813: T16.K 35.37,12.51 C4.+ 35.37,8 33.27,5.91 R30.1 R29.1
N$77  (1 unrouted)
  Top 0.813: R1.1 52.45,80.26
N$78
  Top 0.813: R1.2 T1.B
N$79  (1 unrouted)
  Top 0.813: T11.E 18.61,75.95 T12.E
N$80
  Top 0.813: R11.1 63.44,77.28 63.44,83.18 R6.1 66.42,83.18 66.8,82.8 T1.K
N$81
  Top 0.813: U$8.P$1 T7.K
N$82
  Top 0.813: R2.1 33.72,80.33 32.58,79.18 U$2.P$1
N$83
  Top 0.813: T2.B R2.2
N$84
  pour Top: 0,88.46 0,63.44 70.93,63.44 70.93,88.46
N$85
  Top 0.813: R12.1 43.69,77.41 43.69,83.18 R7.1 47.12,83.18 47.43,82.87 T2.K
N$86
  Top 0.813: T8.K U$9.P$1
N$87
  Top 0.813: U$3.P$1 R3.1
N$88
  Top 0.813: R3.2 T3.B
N$90
  Top 0.813: R13.1 63.31,74.36 63.31,68.45 R8.1 66.48,68.45 66.87,68.83 T3.K
N$91
  Top 0.813: T9.K U$11.P$1
N$92
  Top 0.813: R4.1 35.12,72.14 32.2,72.14 U$4.P$1
N$93
  Top 0.813: R4.2 T4.B
N$95
  Top 0.813: R14.1 43.69,74.36 43.69,68.52 R9.1 47.05,68.52 47.43,68.9 T4.K
N$96
  Top 0.813: U$13.P$1 T10.K
N$97
  Top 0.813: U$5.P$1 27.69,64.77 R5.1
N$98
  Top 0.813: 22.67,71.5 R5.2 22.67,71.5 | 22.67,71.5 T5.B
N$99  (3 unrouted)
  Top 0.813: R6.2 58.1,83.18 T7.E 55.63,86.36 | R8.2 58.1,68.45 T9.E | T8.E 38.42,83.18 R7.2 33.15,83.18 32.07,82.11 T6.E | T10.E 38.42,68.52 R9.2 35.81,65.6 U$7.P$1 | T6.E 22.73,82.11 R10.2 | T6.E U$6.P$1
N$100  (via drill 0.6 pad 2.18)
  other vias: 117.28,52.77
N$101  (via drill 0.6 pad 2.18)
  other vias: 113.73,49.21
N$103  (via drill 0.6 pad 2.18)
  other vias: 104.39,49.78
N$104  (via drill 0.6 pad 2.18)
  other vias: 98.17,49.85
N$105  (via drill 0.6 pad 2.18)
  other vias: 101.28,48.32
N$106  (via drill 0.6 pad 2.18)
  other vias: 94.93,48.45
N$107  (via drill 0.6 pad 2.18)
  other vias: 91.82,49.85
N$108  (via drill 0.6 pad 2.18)
  other vias: 88.58,48.45
N$109  (via drill 0.6 pad 2.18)
  other vias: 85.47,45.4
N$110  (via drill 0.6 pad 2.18)
  other vias: 85.47,47.94
N$111  (via drill 0.6 pad 2.18)
  other vias: 85.47,42.86
N$112  (via drill 0.6 pad 2.18)
  other vias: 85.47,52.39
N$113  (via drill 0.6 pad 2.18)
  other vias: 85.47,54.93
N$114  (via drill 0.6 pad 2.18)
  other vias: 88.58,58.61
N$115  (via drill 0.6 pad 2.18)
  other vias: 91.82,52.39
N$116  (via drill 0.6 pad 2.18)
  other vias: 85.47,49.85
N$117  (via drill 0.6 pad 2.18)
  other vias: 98.17,52.39
N$118  (via drill 0.6 pad 2.18)
  other vias: 98.17,54.93
N$119  (via drill 0.6 pad 2.18)
  other vias: 91.82,54.93
N$120  (via drill 0.6 pad 2.18)
  other vias: 94.93,58.61
N$121  (via drill 0.6 pad 2.18)
  other vias: 104.39,52.39
N$122  (via drill 0.6 pad 2.18)
  other vias: 104.39,54.93
N$123  (via drill 0.6 pad 2.18)
  other vias: 107.51,58.61
N$124  (via drill 0.6 pad 2.18)
  other vias: 110.68,52.39
N$125  (via drill 0.6 pad 2.18)
  other vias: 110.68,54.93
N$126  (via drill 0.6 pad 2.18)
  other vias: 101.28,58.48
N$127  (via drill 0.6 pad 2.18)
  other vias: 113.79,59.44
N$128
  Top 0.813: R34.2 26.92,17.84 28.32,19.24 29.53,19.24 30.99,20.7 T17.B
N$129
  Top 0.813: R29.2 37.85,2.1 37.85,11.56 C3.- 40.58,17.08 T16.B
N$130
  Top 0.813: 43.69,12.19 R26.2 | C3.+ 43.69,9.02 | 43.69,9.02 43.69,12.19 | 43.69,9.02 47.37,9.02 49.15,7.24 R25.2 | T15.K 43.69,12.19
N$131
  Top 0.813: C2.- 49.15,9.91 R25.1 46.1,17.08 T15.B
N$132
  Top 0.813: C2.+ U$18.P$1 58.61,14.35 R23.2
N$134  (via drill 0.5 pad 2.18)
  other vias: 33.59,22.86
N$135  (via drill 0.5 pad 2.18)
  other vias: 37.4,19.69
N$136
  Top 0.813: U$29.P$1 104.14,14.29 105.86,12.57 131,12.57 135.7,17.27 145.54,17.27 154.81,8 U$30.P$1
N$137  (via drill 0.5 pad 2.18)
  other vias: 37.4,17.08
N$138  (via drill 0.5 pad 2.18)
  other vias: 40.51,11.62
N$139
  Top 0.813: C1.+ 51.88,17.08 R23.1 51.88,13.02 R22.2
N$140  (via drill 0.6 pad 2.54)
  other vias: 86.55,8
N$141
  Top 0.813: R30.2 45.78,5.52 R26.1 R24.2 61.28,2.03 61.28,10.99 R22.1 64.07,16.7 59.44,16.7 59.44,22.35 C7.+ 55.05,22.35 54.55,22.86 D1.A
N$142  (via drill 0.5 pad 2.18)
  other vias: 33.53,14.6
N$143
  Top 0.813: R32.1 30.61,16.76 C8.1 T17.E U$19.P$1 | U$19.P$1 T16.E | U$19.P$1 D1.C 43.69,22.86 T15.E C1.- 53.47,19.62 54.29,18.8 C7.-
N$145  (via drill 0.5 pad 2.18)
  other vias: 41.27,22.86
N$146
  Top 0.813: U$20.P$1 R24.1
N$148  (via drill 0.5 pad 2.18)
  other vias: 64.07,10.99
N$149
  Top 0.813: U$37.P$1 T17.K
N$150  (via drill 0.5 pad 2.18)
  other vias: 43.69,19.69
N$151  (via drill 0.5 pad 2.18)
  other vias: 43.75,17.08
N$152  (via drill 0.5 pad 2.18)  (1 unrouted)
  other vias: 57.28,22.35 51.44,22.86
N$155  (via drill 0.5 pad 2.18)
  other vias: 57.28,18.8
N$156  (via drill 0.5 pad 2.18)
  other vias: 61.85,14.29
N$157  (via drill 0.5 pad 2.18)
  other vias: 49.78,19.69
N$158  (via drill 0.5 pad 2.18)
  other vias: 53.91,10.99
N$159  (via drill 0.5 pad 2.18)
  other vias: 51.88,14.35
N$160  (via drill 0.5 pad 2.18)
  other vias: 49.09,14.03
N$161  (via drill 0.5 pad 2.18)
  other vias: 45.78,12.19
N$162  (via drill 0.5 pad 2.18)
  other vias: 43.69,14.54
N$163  (via drill 0.5 pad 2.18)
  other vias: 30.99,22.86
N$164  (via drill 0.5 pad 2.18)
  other vias: 28.45,22.86
N$165  (via drill 0.5 pad 2.18)
  other vias: 25.34,17.78
N$166  (via drill 0.5 pad 2.18)
  other vias: 37.4,14.54
N$167  (via drill 0.5 pad 2.18)
  other vias: 53.91,2.03
N$168  (via drill 0.5 pad 2.18)
  other vias: 55.25,6.48
N$169  (via drill 0.5 pad 2.18)
  other vias: 49.15,3.94
N$170  (via drill 0.5 pad 2.18)
  other vias: 52.51,6.48
N$171  (via drill 0.5 pad 2.18)
  other vias: 45.78,2.03
N$172  (via drill 0.5 pad 2.18)
  other vias: 43.05,2.1
N$173  (via drill 0.5 pad 2.18)
  other vias: 25.34,7.68
N$174  (via drill 0.5 pad 2.18)
  other vias: 29.34,6.6
N$175  (via drill 0.5 pad 2.18)
  other vias: 32.83,5.52
N$176  (via drill 0.5 pad 2.18)
  other vias: 32.89,2.1
N$177  (via drill 0.5 pad 2.18)
  other vias: 43.05,5.52
N$178  (via drill 0.5 pad 2.18)
  other vias: 35.43,10.29
N$179  (via drill 0.5 pad 2.18)
  other vias: 29.34,16.76
N$180  (via drill 0.5 pad 2.18)
  other vias: 33.53,19.62
N$181  (via drill 0.5 pad 2.18)
  other vias: 32.7,10.35
N$182  (via drill 0.5 pad 2.18)
  other vias: 40.58,8.95
N$183  (via drill 0.5 pad 2.18)
  other vias: 49.78,17.02
N$184
  Top 0.813: R10.1 R15.1 26.23,76.58 T5.K
N$185
  Top 0.813: U$14.P$1 33.15,87.19 T6.K
N$186
  Top 0.813: R16.1 U$16.P$1
N$187
  Top 0.813: T11.B R16.2
N$189
  Top 0.813: T11.K 17.02,82.87 16.51,83.38 R18.1 12.95,83.38 12.95,77.41 R20.1
N$190
  Top 0.813: T13.K U$21.P$1
N$191
  Top 0.813: R17.1 U$17.P$1
N$192
  Top 0.813: T12.B R17.2
N$193  (1 unrouted)
  Top 0.813: R19.2 7.87,68.39 T14.E | R18.2 7.87,83.38 T13.E 3.36,86.49 U$22.P$1
N$194
  Top 0.813: T12.K 16.83,68.9 16.32,68.39 R19.1 12.95,68.39 12.95,74.55 R21.1
N$195
  Top 0.813: T14.K U$23.P$1
N$196  (2 unrouted)
  Top 0.813: T1.E U$12.P$1 T3.E | T2.E U$10.P$1 T4.E | U$15.P$1 31.18,68.96 T5.E
N$221  (via drill 0.6 pad 2.18)
  other vias: 55.5,80.26
N$231  (via drill 0.6 pad 2.18)
  other vias: 55.5,83.19
N$232  (via drill 0.6 pad 2.18)
  other vias: 68.64,68.83
N$233  (via drill 0.6 pad 2.18)
  other vias: 55.5,68.45
N$234  (via drill 0.6 pad 2.18)
  other vias: 55.5,71.37
N$235  (via drill 0.6 pad 2.18)
  other vias: 65.66,71.37
N$236  (via drill 0.6 pad 2.18)
  other vias: 55.5,77.28
N$237  (via drill 0.6 pad 2.18)
  other vias: 68.64,73.91
N$238  (via drill 0.6 pad 2.18)
  other vias: 65.6,77.28
N$239  (via drill 0.6 pad 2.18)
  other vias: 45.97,68.52
N$240  (via drill 0.6 pad 2.18)
  other vias: 65.66,68.39
N$241  (via drill 0.6 pad 2.18)
  other vias: 63.18,65.41
N$242  (via drill 0.6 pad 2.18)
  other vias: 68.64,71.37
N$243  (via drill 0.6 pad 2.18)
  other vias: 65.66,74.36
N$244  (via drill 0.6 pad 2.18)
  other vias: 55.5,74.36
N$245  (via drill 0.6 pad 2.18)
  other vias: 65.66,83.19
N$246  (via drill 0.6 pad 2.18)
  other vias: 68.71,82.8
N$247  (via drill 0.6 pad 2.18)
  other vias: 35.81,71.44
N$248  (via drill 0.6 pad 2.18)
  other vias: 68.64,77.72
N$249  (via drill 0.6 pad 2.18)
  other vias: 65.66,80.26
N$250  (via drill 0.6 pad 2.18)
  other vias: 68.64,80.26
N$251  (via drill 0.6 pad 2.18)
  other vias: 63.18,86.36
N$252  (via drill 0.6 pad 2.18)
  other vias: 58.17,86.36
N$253  (via drill 0.6 pad 2.18)
  other vias: 49.02,80.33
N$254  (via drill 0.6 pad 2.18)
  other vias: 60.71,86.36
N$255  (via drill 0.6 pad 2.18)
  other vias: 43.5,86.42
N$256  (via drill 0.6 pad 2.18)
  other vias: 40.96,86.42
N$257  (via drill 0.6 pad 2.18)
  other vias: 38.42,86.42
N$258  (via drill 0.6 pad 2.18)
  other vias: 35.81,83.19
N$259  (via drill 0.6 pad 2.18)
  other vias: 45.97,71.44
N$260  (via drill 0.6 pad 2.18)
  other vias: 49.02,71.44
N$261  (via drill 0.6 pad 2.18)
  other vias: 5.08,83.38
N$262  (via drill 0.6 pad 2.18)
  other vias: 45.97,83.19
N$263  (via drill 0.6 pad 2.18)
  other vias: 60.64,65.41
N$264  (via drill 0.6 pad 2.18)
  other vias: 45.97,80.33
N$265  (via drill 0.6 pad 2.18)
  other vias: 49.02,73.98
N$266  (via drill 0.6 pad 2.18)
  Top 0.813: v58.1,65.4 54.8,65.4
N$267  (via drill 0.6 pad 2.18)
  other vias: 49.02,68.9
N$268  (via drill 0.6 pad 2.18)
  other vias: 49.02,82.87
N$269  (via drill 0.6 pad 2.18)
  other vias: 49.02,77.79
N$270  (via drill 0.6 pad 2.18)
  other vias: 45.97,77.41
N$271  (via drill 0.6 pad 2.18)
  other vias: 45.97,74.36
N$272  (via drill 0.6 pad 2.18)
  other vias: 40.96,65.47
N$273  (via drill 0.6 pad 2.18)
  other vias: 35.81,68.52
N$274  (via drill 0.6 pad 2.18)
  other vias: 25.72,87.25
N$275  (via drill 0.6 pad 2.18)
  other vias: 38.42,65.47
N$276  (via drill 0.6 pad 2.18)
  other vias: 15.24,71.44
N$277  (via drill 0.6 pad 2.18)
  other vias: 35.81,80.33
N$278  (via drill 0.6 pad 2.18)
  other vias: 35.81,74.36
N$279  (via drill 0.6 pad 2.18)
  other vias: 35.81,77.41
N$280  (via drill 0.6 pad 2.18)
  other vias: 43.5,65.47
N$281  (via drill 0.6 pad 2.18)
  other vias: 18.61,82.93
N$282  (via drill 0.6 pad 2.18)
  other vias: 18.61,80.33
N$283  (via drill 0.6 pad 2.18)
  other vias: 18.61,77.85
N$284  (via drill 0.6 pad 2.18)
  other vias: 15.24,80.33
N$285  (via drill 0.6 pad 2.18)
  other vias: 15.24,83.38
N$286  (via drill 0.6 pad 2.18)
  other vias: 12.89,86.55
N$287  (via drill 0.6 pad 2.18)
  other vias: 10.41,86.55
N$288  (via drill 0.6 pad 2.18)
  other vias: 7.87,86.49
N$289  (via drill 0.6 pad 2.18)
  other vias: 5.08,80.33
N$290  (via drill 0.6 pad 2.18)
  other vias: 5.08,77.41
N$291  (via drill 0.6 pad 2.18)
  other vias: 5.08,74.55
N$292  (via drill 0.6 pad 2.18)
  other vias: 7.87,65.6
N$293  (via drill 0.6 pad 2.18)
  other vias: 10.41,65.6
N$294  (via drill 0.6 pad 2.18)
  other vias: 139.45,38.67
N$295  (via drill 0.6 pad 2.18)
  other vias: 15.18,68.39
N$296  (via drill 0.6 pad 2.18)
  other vias: 5.02,68.39
N$297  (via drill 0.6 pad 2.18)
  other vias: 15.24,77.41
N$298  (via drill 0.6 pad 2.18)
  other vias: 12.95,65.53
N$299  (via drill 0.6 pad 2.18)
  other vias: 144.53,38.67
N$300  (via drill 0.6 pad 2.18)
  other vias: 147.32,38.42
N$301  (via drill 0.6 pad 2.18)
  other vias: 153.61,58.8
N$302  (via drill 0.6 pad 2.18)
  other vias: 147.19,58.67
N$303  (via drill 0.6 pad 2.18)
  other vias: 153.61,48.64
N$304  (via drill 0.6 pad 2.18)
  other vias: 156.91,50.04
N$305  (via drill 0.6 pad 2.18)
  other vias: 150.43,49.97
N$306  (via drill 0.6 pad 2.18)
  other vias: 147.19,48.51
N$307  (via drill 0.6 pad 2.18)
  other vias: 140.84,49.66
N$308  (via drill 0.6 pad 2.18)
  other vias: 144.02,49.91
N$309  (via drill 0.6 pad 2.18)
  other vias: 144.02,52.51
N$310  (via drill 0.6 pad 2.18)
  other vias: 150.37,52.51
N$311  (via drill 0.6 pad 2.18)
  other vias: 156.91,52.51
N$312  (via drill 0.6 pad 2.18)
  other vias: 156.91,55.05
N$313  (via drill 0.6 pad 2.18)
  other vias: 150.3,55.05
N$314  (via drill 0.6 pad 2.18)
  other vias: 144.08,55.05
N$315  (via drill 0.6 pad 2.18)
  other vias: 140.84,59.75
N$316  (via drill 0.6 pad 2.18)
  other vias: 107.51,48.45
N$317  (via drill 0.6 pad 2.18)
  other vias: 92.71,43.31
N$318  (via drill 0.6 pad 2.18)
  other vias: 135.32,44.32
N$319  (via drill 0.6 pad 2.18)
  other vias: 135.32,41.66
N$320  (via drill 0.6 pad 2.18)
  other vias: 132.33,41.72
N$321  (via drill 0.6 pad 2.18)
  other vias: 119.63,41.72
N$322  (via drill 0.6 pad 2.18)
  other vias: 124.4,22.86
N$323  (via drill 0.6 pad 2.18)
  other vias: 102.87,43.31
N$324  (via drill 0.6 pad 2.18)
  other vias: 138.75,12.7
N$325  (via drill 0.6 pad 2.18)
  other vias: 142.49,12.7
N$326  (via drill 0.6 pad 2.18)
  other vias: 110.68,49.78
N$327  (via drill 0.6 pad 2.18)
  other vias: 146.3,12.76
N$328  (via drill 0.6 pad 2.18)
  other vias: 145.1,7.94
N$329  (via drill 0.6 pad 2.18)
  other vias: 146.3,22.86
N$330  (via drill 0.6 pad 2.18)
  other vias: 142.49,22.86
N$331  (via drill 0.6 pad 2.18)
  other vias: 138.68,22.86
N$332  (via drill 0.6 pad 2.18)
  other vias: 134.56,22.86
N$333  (via drill 0.6 pad 2.18)
  other vias: 155.96,15.56
N$334  (via drill 0.6 pad 2.18)
  other vias: 124.4,19.05
N$335  (via drill 0.6 pad 2.18)
  other vias: 166.31,19.69
N$336  (via drill 0.6 pad 2.18)
  other vias: 138.62,8
N$337  (via drill 0.6 pad 2.18)
  other vias: 93.09,8
N$338  (via drill 0.6 pad 2.18)
  other vias: 112.59,8.06
N$339  (via drill 0.6 pad 2.18)
  other vias: 119.13,7.94
N$340
  Top 0.813: T6.B 25.72,84.65 R15.2
N$341
  Top 0.813: R14.2 40.96,74.36 T10.B
N$342
  Top 0.813: R13.2 60.64,74.36 T9.B
N$343
  Top 0.813: R11.2 60.64,77.28 T7.B
N$344
  Top 0.813: R12.2 40.96,77.41 T8.B
N$345
  Top 0.813: R21.2 10.41,74.55 T14.B
N$346
  Top 0.813: T13.B 10.41,77.41 R20.2
U$34
  pour Top: 23.24,25.4 65.53,25.4 65.53,0.38 23.24,0.38
(copper drawn outside any net)
  shapes: Top area x82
